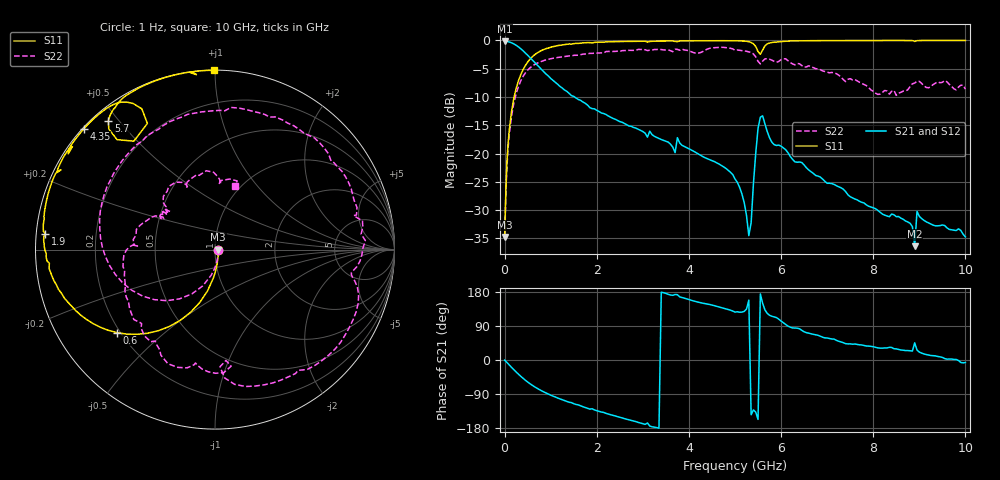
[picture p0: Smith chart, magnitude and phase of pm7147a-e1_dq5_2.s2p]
# GHz S DB R 50
! S-Parameters data
! Freq  dbS11  angS11  dbS21  angS21  dbS12  angS12  dbS22  angS22
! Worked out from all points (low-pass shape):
!   279 points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, 1 Hz to 10 GHz, reference 50 ohm
!   highest |S21| = -0.16 dB at 7.943 kHz (marker M1); lowest = -36.4 dB at 8.9 GHz (marker M2)
!   |S21| within 3 dB of the highest: start of sweep to 564.4 MHz
!   lowest |S11| = -34.8 dB at 7.943 kHz (marker M3), VSWR 1.04, Z = 51.9 - j0.00121 ohm
!   |S11| at or under -10 dB: start of sweep to 207.1 MHz
!   |S22| runs from -34.8 to -1.2 dB; largest |S21 - S12| = 1.7e-12
!   S11 on the Smith chart (normalised r, x): 1 Hz: 1.04, -0.00; 600 MHz: 0.19, -0.35; 1.9 GHz: 0.03, +0.05; 4.35 GHz: 0.00, +0.39; 5.7 GHz: 0.04, +0.47; 10 GHz: 0.00, +0.99
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1e-09  -34.76 -0.0  -0.16 0.0  -0.16 0.0  -34.76 -0.0
7.9433e-06  -34.76 -0.0  -0.16 -0.0  -0.16 -0.0  -34.76 -0.0
0.05011872  -21.72 -81.9  -0.19 -6.5  -0.19 -6.5  -22.46 -83.7
0.15  -12.58 -100.3  -0.42 -19.3  -0.42 -19.3  -13.40 -108.7
0.6  -2.90 -139.8  -3.46 -66.8  -3.46 -66.8  -4.53 -171.3
1.05  -1.09 -162.2  -7.07 -95.4  -7.07 -95.4  -3.15 149.9
1.7  -0.44 179.0  -10.89 -123.3  -10.89 -123.3  -2.43 109.6
1.9  -0.45 174.6  -12.06 -128.7  -12.06 -128.7  -2.28 98.0
2.55  -0.19 162.7  -14.47 -152.8  -14.47 -152.8  -1.81 65.6
3.35  -0.11 150.6  -17.33 -179.8  -17.33 -179.8  -1.59 26.5
4.35  -0.06 137.4  -20.74 148.8  -20.74 148.8  -1.73 -14.7
5.05  -0.07 127.8  -25.09 127.4  -25.09 127.4  -1.69 -57.1
5.3  -0.23 122.5  -34.51 157.9  -34.51 157.9  -2.02 -73.5
5.5  -1.97 118.2  -15.55 -156.7  -15.55 -156.7  -3.70 -87.6
5.7  -0.61 129.6  -16.12 123.1  -16.12 123.1  -3.23 -89.7
6.7  -0.04 115.6  -23.52 67.7  -23.52 67.7  -4.80 -146.0
7.65  -0.02 107.0  -28.18 41.0  -28.18 41.0  -7.15 162.1
8.35  -0.01 101.5  -31.17 33.5  -31.17 33.5  -9.50 143.7
8.8  -0.01 98.0  -32.33 24.4  -32.33 24.4  -8.15 137.7
8.9  -0.17 96.1  -36.38 45.3  -36.38 45.3  -7.53 129.5
8.95  -0.04 97.9  -30.21 26.2  -30.21 26.2  -7.21 126.1
10  -0.00 90.3  -34.73 -6.6  -34.73 -6.6  -8.61 72.2
